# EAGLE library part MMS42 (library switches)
4PDT - SWITCH SLIDE 4PDT 300MA 30V
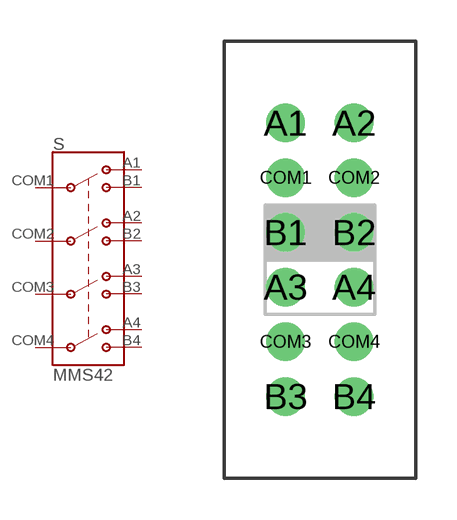
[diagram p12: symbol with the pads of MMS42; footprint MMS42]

Designator prefix S

## MMS42 (DIGIKEY: 679-1858-ND; MPN: MMS42)  [MMS42]
A1  1TA
A2  2TA
A3  3TA
A4  4TA
B1  1TB
B2  2TB
B3  3TB
B4  4TB
COM1  1P
COM2  2P
COM3  3P
COM4  4P

## Footprint MMS42 (pad centres in mm)
MMS42 - 4P2T Drawn from http://www.apem.com/files/apem/brochures/MMS_MICRO_SLIDE.pdf DigiKey: 679-1858-ND
drill 0.9: A1 -1.25,5; A2 1.25,5; A3 -1.25,-1; A4 1.25,-1; B1 -1.25,1; B2 1.25,1; B3 -1.25,-5; B4 1.25,-5; COM1 -1.25,3; COM2 1.25,3; COM3 -1.25,-3; COM4 1.25,-3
